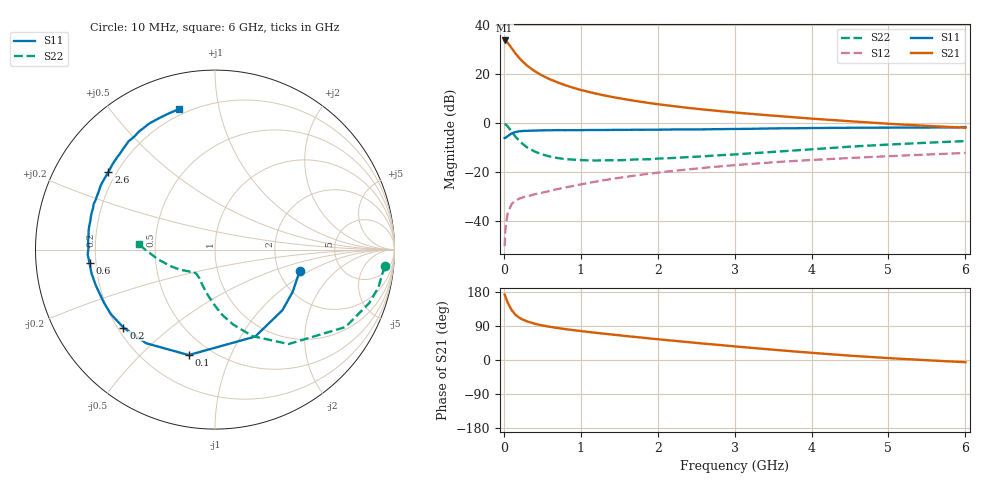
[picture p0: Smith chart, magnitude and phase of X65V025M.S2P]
! SIEMENS Small Signal Semiconductors
! BFP193W
! Si NPN RF Bipolar Junction Transistor in SOT343
! VCE = 5 V  IC = 25 mA
! Common Emitter S-Parameters:  April 1994
# GHz  S  MA  R  50
!  f  S11  S21  S12  S22
! GHz  MAG  ANG  MAG  ANG  MAG  ANG  MAG  ANG
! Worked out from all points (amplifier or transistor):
!   40 points, 10 MHz to 6 GHz, reference 50 ohm
!   highest |S21| = 33.7 dB at 10 MHz (marker M1)
!   |S21| within 3 dB of that: start of sweep to 98.29 MHz
!   unconditionally stable (mu >= 1): 886.5 MHz to 4.145 GHz
!   at 200 MHz: K = 0.39, MSG = 28.8 dB, |S12| = -31.1 dB
!   at 1.5 GHz: K = 1.11, MAG = 14.3 dB, |S12| = -22.5 dB
!   at 6 GHz: K = 0.93, MSG = 5.2 dB, |S12| = -12.3 dB
!   S11 on the Smith chart (normalised r, x): 10 MHz: 2.60, -0.82; 100 MHz: 0.38, -0.71; 200 MHz: 0.22, -0.35; 600 MHz: 0.17, -0.05; 2.6 GHz: 0.17, +0.32; 6 GHz: 0.17, +0.76
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0.01  0.4872 -14.3  48.33 172.8  0.003 86.3  0.949 -5.6
0.02  0.4926 -28.6  47.78 167.8  0.0062 78.2  0.9346 -13.0
0.03  0.5051 -41.9  46.7 162.1  0.009 75.3  0.909 -19.2
0.05  0.5338 -65.2  43.3 151.4  0.0141 66.3  0.8451 -30.7
0.1  0.6055 -104.0  33.93 132.1  0.0217 52.2  0.6669 -52.1
0.15  0.6475 -126.3  26.41 119.5  0.0257 44.8  0.5253 -66.6
0.2  0.6698 -139.6  21.14 111.7  0.028 41.3  0.4292 -76.4
0.25  0.6824 -148.2  17.58 106.1  0.03 40.7  0.365 -83.8
0.3  0.6861 -154.5  14.86 102.0  0.0313 40.3  0.3158 -89.6
0.4  0.6937 -163.5  11.41 95.8  0.0345 42.0  0.259 -98.5
0.5  0.7008 -169.3  9.244 91.2  0.0373 44.0  0.2256 -105.5
0.6  0.703 -173.9  7.745 87.5  0.0405 46.2  0.204 -111.0
0.8  0.7048 179.1  5.865 81.5  0.0476 50.3  0.1814 -118.7
1.1  0.7121 171.5  4.306 74.0  0.0589 53.6  0.1704 -126.6
1.3  0.7126 166.9  3.646 69.4  0.0671 54.8  0.1708 -129.9
1.6  0.7179 161.2  2.991 62.9  0.0791 55.6  0.1737 -133.7
2.2  0.7305 150.6  2.198 50.9  0.1036 54.7  0.1908 -141.1
2.6  0.7344 143.9  1.867 43.2  0.12 52.9  0.2065 -145.9
3.2  0.7533 134.5  1.53 32.4  0.1438 49.6  0.2371 -153.4
4.5  0.7924 117.5  1.077 11.4  0.1907 41.1  0.3252 -170.7
5.5  0.8013 108.6  0.866 -0.6  0.2244 34.9  0.3916 179.7
6  0.8086 104.3  0.792 -5.9  0.2418 32.1  0.4232 176.1
